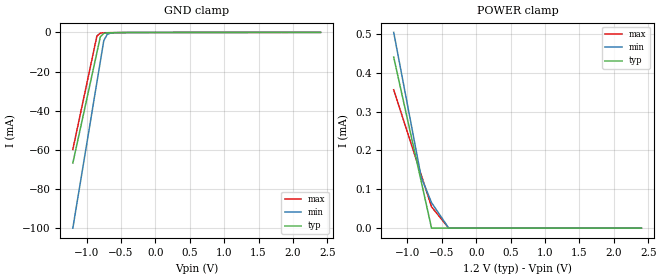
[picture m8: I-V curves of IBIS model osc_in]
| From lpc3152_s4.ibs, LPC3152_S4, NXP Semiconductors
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[Model] osc_in
Model_type Input
Vinl = 360.000mV
Vinh = 840.000mV
C_comp .836pF .820pF .842pF
| variable typ   min   max
[Voltage Range] 1.20000V 1.10000V 1.30000V
[POWER Clamp Reference] 1.20000V 1.10000V 1.30000V
[GND Clamp Reference] 0.00000V 0.00000V 0.00000V
[Temperature Range]   25   85   -40
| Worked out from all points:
|   GND clamp passes 1 mA (typ) near -0.77 V on its own axis
[GND Clamp]
-1.2V     -66.69mA   -99.89mA   -59.74mA
-850mV    -10.27mA   -25.43mA   -1.794mA
-800mV    -2.215mA   -14.79mA   -356.5uA
-750mV    -460.4uA   -4.15mA    -156.1uA
-700mV    -165.2uA   -981.9uA   -137.6uA
-650mV    -144.1uA   -302.6uA   -119uA
-600mV    -123uA     -119.4uA   -100.5uA
-375mV    -27.94uA   -42.56uA   -17.03uA
-350mV    -17.39uA   -34.02uA   -16.6uA
-300mV    -16.35uA   -16.95uA   -15.73uA
2.4V      39.53uA    32.2uA     30.97uA
[POWER Clamp]
-1.2V     440uA      503.8uA    355.9uA
-800mV    120uA      130.9uA    136.9uA
-650mV    0A         65.46uA    54.76uA
-400mV    0A         0A         0A
2.4V      0A         0A         0A
